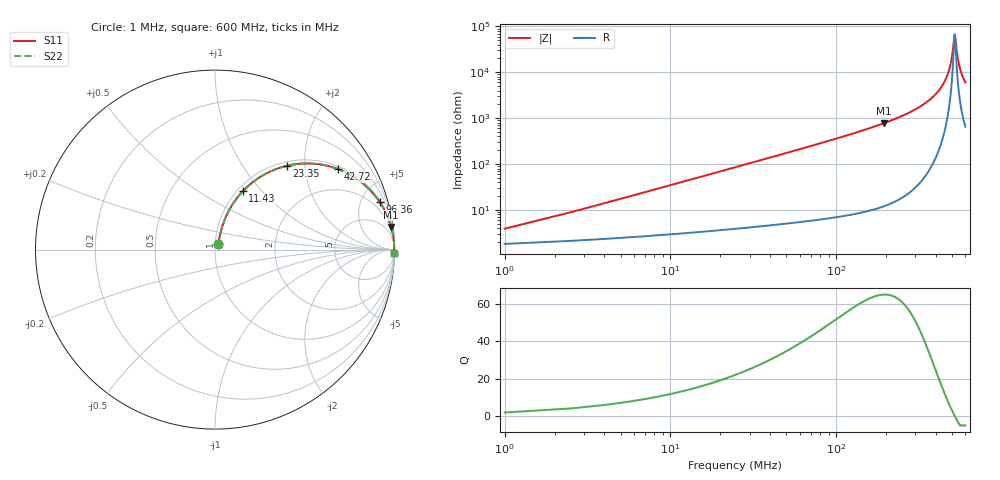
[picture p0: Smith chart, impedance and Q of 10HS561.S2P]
! Coilcraft 1008HS-561 Chip Inductor
! 02 July 2002
# MHZ S MA R 50
!Freq  MagS11  AngS11  MagS21  AngS21  MagS12  AngS12  MagS22  AngS22
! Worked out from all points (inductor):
!   404 points, 1 MHz to 600 MHz, reference 50 ohm
!   read as one part in series: L = 550 nH near 3.98 MHz
!   highest Q = 64.8 at 193.2 MHz (marker M1), where L = 639 nH
!   self-resonance near 516.5 MHz
!   S11 on the Smith chart (normalised r, x): 1 MHz: 1.04, +0.07; 11.43 MHz: 1.06, +0.79; 23.35 MHz: 1.08, +1.62; 42.72 MHz: 1.09, +2.97; 96.36 MHz: 1.14, +6.90; 600 MHz: open
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1  0.03833 60.3  0.9816 -1.9  0.9816 -1.9  0.03833 60.3
6.96  0.2295 70.5  0.9483 -13.2  0.9483 -13.2  0.2295 70.5
11.43  0.3591 64.6  0.906 -21.0  0.906 -21.0  0.3591 64.6
23.35  0.6152 49.4  0.76 -37.9  0.76 -37.9  0.6152 49.4
42.72  0.8179 33.3  0.55 -54.8  0.55 -54.8  0.8179 33.3
65.07  0.908 23.4  0.3973 -65.2  0.3973 -65.2  0.908 23.4
96.36  0.9554 16.1  0.2769 -72.8  0.2769 -72.8  0.9554 16.1
102.32  0.9604 15.1  0.2609 -73.8  0.2609 -73.8  0.9604 15.1
193.21  0.9899 7.3  0.1276 -81.8  0.1276 -81.8  0.9899 7.3
202.15  0.9909 6.9  0.1202 -82.2  0.1202 -82.2  0.9909 6.9
301.98  0.9968 3.6  0.06299 -85.2  0.06299 -85.2  0.9968 3.6
401.81  0.9984 1.6  0.02858 -85.9  0.02858 -85.9  0.9984 1.6
437.57  0.9985 1.1  0.01887 -85.0  0.01887 -85.0  0.9985 1.1
465.88  0.9986 0.7  0.01184 -82.8  0.01184 -82.8  0.9986 0.7
486.74  0.9986 0.4  0.006996 -78.1  0.006996 -78.1  0.9986 0.4
501.64  0.9986 0.2  0.003772 -67.3  0.003772 -67.3  0.9986 0.2
513.56  0.9985 0.0  0.001713 -30.2  0.001713 -30.2  0.9985 0.0
518.03  0.9985 -0.0  0.001497 3.9  0.001497 3.9  0.9985 -0.0
535.91  0.9984 -0.2  0.00419 68.0  0.00419 68.0  0.9984 -0.2
549.32  0.9984 -0.4  0.006841 76.1  0.006841 76.1  0.9984 -0.4
571.67  0.9982 -0.6  0.01124 80.7  0.01124 80.7  0.9982 -0.6
600  0.9981 -0.9  0.01665 82.8  0.01665 82.8  0.9981 -0.9
